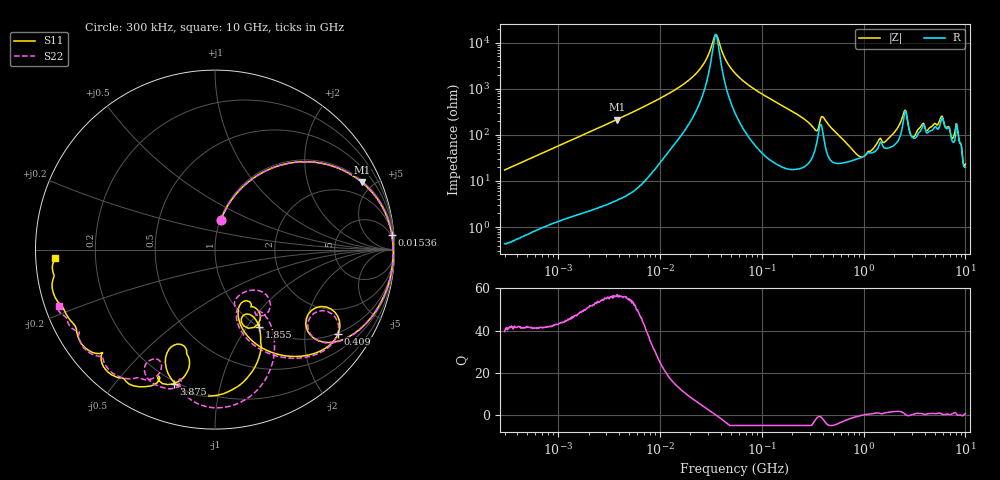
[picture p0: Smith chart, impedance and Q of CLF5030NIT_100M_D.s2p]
! S-Parameter Data Generated by TDK Corporation
! Copyright(C) 2019 TDK Corporation.
! All Rights Reserved.
! TDK P/N: CLF5030NIT-100M-D (Inductor)
! Property: L=10uH at 100kHz
! Size(LxWxT): 5.3x5x2.7mm
! Model Type: s2p (Touchstone File Format Version 1.0)
! Frequency: DC=Yes Start=0.3MHz Stop=10000MHz 802points Log-sweep
! Model Generated on May 10, 2019
! Port Assignments:
!  1 ---@@@--- 2
! Applicable Conditions:
!  Temperature = 25 degC
!  DC Bias Current = 0 A
!  Small Signal Operation
! Terms and conditions regarding TDK Simulation Models
! (1)This simulation model is being provided solely for informational purposes. Please refer to the specifications of the products in terms of detailed characteristics of such products.
! (2)In no event shall TDK Corporation of any of its subsidiaries be liable for any loss or damage arising, directly or indirectly,
!  From any information contained in this simulation model, including, but not limited to loss or damages arising from any inaccuracies, omissions or errors in connection with such information.
! (3)Any and all copyrights on this simulation model are owned by TDK Corporation.
!  Duplication or redistribution of this simulation model without prior written permission from TDK Corporation is prohibited.
! (4)This simulation model is subject to any modification or change without any prior notice.
! (5)Neither TDK Corporation nor any of its subsidiaries shall make any warranty, express or implied,
!  Including but not limited to the correctness, implied warranties of merchantability and fitness for a particular purpose with respect to this simulation models.
! (6)The use of this simulation model shall be deemed to have consented to the terms and conditions hereof.
# Hz S MA R 50
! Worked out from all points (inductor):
!   801 points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, 300 kHz to 10 GHz, reference 50 ohm
!   read as one part in series: L = 9.17 uH near 318.3 kHz
!   highest Q = 56.3 at 3.777 MHz (marker M1), where L = 9.02 uH
!   self-resonance near 35.12 MHz
!   S11 on the Smith chart (normalised r, x): 300 kHz: 1.01, +0.35; 15.36 MHz: 3, +24; 409 MHz: 0.98, -2.95; 1.855 GHz: 1.00, -1.14; 3.875 GHz: 0.19, -0.72; 10 GHz: 0.06, -0.03
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300000  0.1706 78.8  0.9809 -9.8  0.9808 -9.8  0.1706 78.9
1713600  0.6887 45.3  0.7111 -43.6  0.7111 -43.6  0.6887 45.3
3777497  0.8998 24.7  0.4206 -64.3  0.4206 -64.3  0.8999 24.7
9671944  0.9799 9.2  0.166 -78.7  0.166 -78.7  0.9799 9.1
1.535588e7  0.9885 4.7  0.09285 -80.9  0.09287 -80.9  0.9885 4.7
2.567637e7  0.9924 0.8  0.03361 -77.2  0.03363 -77.2  0.9924 0.8
3.555278e7  0.9933 -1.4  0.006622 -1.0  0.006626 -1.0  0.9933 -1.5
5.477226e7  0.9926 -4.8  0.04552 77.3  0.04553 77.3  0.9927 -4.9
3.126428e8  0.7928 -40.5  0.4731 38.4  0.4731 38.4  0.7967 -40.5
4.089972e8  0.8305 -34.3  0.3363 35.4  0.3362 35.4  0.8351 -36.0
5.580434e8  0.7183 -55.7  0.5652 22.4  0.5652 22.3  0.7157 -57.2
8.643532e8  0.4522 -71.1  0.6893 -12.0  0.6893 -12.0  0.4423 -72.8
1.24442e9  0.3788 -57.1  0.6553 -44.4  0.6553 -44.4  0.2867 -58.1
1.767019e9  0.4528 -59.8  0.5514 -77.0  0.5515 -77.0  0.4398 -53.2
1.854885e9  0.4967 -60.3  0.5236 -84.4  0.5237 -84.4  0.4769 -52.8
2.568366e9  0.8153 -98.4  0.1214 -96.7  0.1218 -96.8  0.8765 -84.5
3.093017e9  0.5665 -111.7  0.2939 -91.0  0.2935 -91.1  0.7595 -105.3
3.874538e9  0.7824 -107.1  0.1448 -113.8  0.145 -114.1  0.8085 -118.0
4.749267e9  0.8682 -118.3  0.1524 -132.2  0.152 -132.4  0.7465 -114.2
7.316673e9  0.8905 -150.1  0.07741 -144.2  0.07664 -144.1  0.8854 -148.7
8.546531e9  0.9327 -165.1  0.02728 -123.1  0.02714 -123.0  0.9152 -156.1
1e10  0.8904 -177.0  0.04611 -120.3  0.04636 -120.5  0.9223 -160.0
